{attribute 'qualified_only'}
{attribute 'strict'}
(* Condition node with EXTENDS and multiple interface check *)
FUNCTION_BLOCK FB_ConditionNode EXTENDS FB_BaseNode
VAR_INPUT
    bCondition : BOOL;
END_VAR
VAR
    _bLastCondition : BOOL;
    _nEvaluationCount : UDINT;
END_VAR

METHOD Tick : E_NodeStatus
_nEvaluationCount := _nEvaluationCount + 1;
_bLastCondition := bCondition;

IF bCondition THEN
    Tick := E_NodeStatus.SUCCESS;
    SetProgressComplete();
ELSE
    Tick := E_NodeStatus.FAILURE;
END_IF

eLastStatus := Tick;
END_METHOD

METHOD Reset : BOOL
SUPER^.Reset();
_bLastCondition := FALSE;
_nEvaluationCount := 0;
Reset := TRUE;
END_METHOD

PROPERTY EvaluationCount : UDINT
GET
EvaluationCount := _nEvaluationCount;
END_GET
END_PROPERTY

PROPERTY LastCondition : BOOL
GET
LastCondition := _bLastCondition;
END_GET
END_PROPERTY

END_FUNCTION_BLOCK
